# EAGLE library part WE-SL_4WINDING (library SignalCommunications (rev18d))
SMD Common-Mode Choke Line Filter WE-SL For distortion-free removal of noise from transmitted electrical signals - 2 or 4 winding configuration - Offering a wide band width with the core materials of NiZn and MnZn -- Current compensated choke for data and signal lines -- USB/CAN/ISDN-Bus -- Power supply systems -- Control lines -- LAN, PBX, cable TV, CD-ROM, 8mm video, etc. Details see: http://katalog.we-online.de/en/pbs/WE-SL? Updated by Dan Xu 2014-07-11 2014 (C) Würth Elektronik
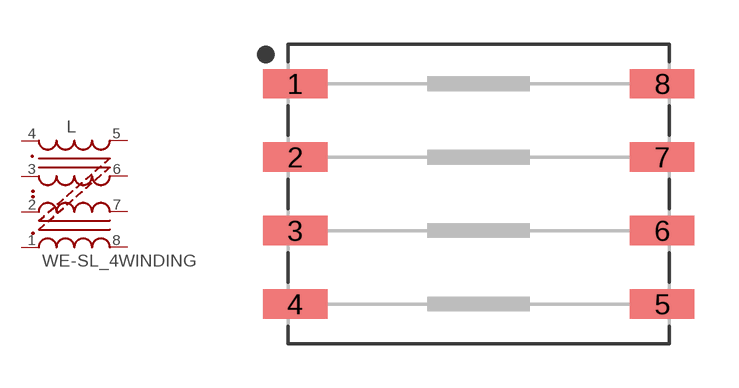
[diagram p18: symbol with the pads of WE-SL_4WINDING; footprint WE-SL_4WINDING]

Designator prefix L

## WE-SL_4WINDING_744201, WE-SL_4WINDING_744202, WE-SL_4WINDING_744203, WE-SL_4WINDING_744204, WE-SL_4WINDING_744205  [WE-SL_4WINDING]
1  4  pas
2  3  pas
3  2  pas
4  1  pas
5  8  pas
6  7  pas
7  6  pas
8  5  pas

## Footprint WE-SL_4WINDING (pad centres in mm)
SMD Common-Mode Line Filter WE-SL
smd 2.2 x 1: 1 -6.25,3.75; 2 -6.25,1.25; 3 -6.25,-1.25; 4 -6.25,-3.75; 5 6.25,-3.75; 6 6.25,-1.25; 7 6.25,1.25; 8 6.25,3.75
